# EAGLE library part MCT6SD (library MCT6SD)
Choice of 3 current transfer ratios; Two isolated channels per package; VDE approved for IEC60747-5-2; Two packages fit into a 16 lead DIP socket; Underwriters Laboratory (U.L.) recognized File E90700 Source: Datasheet
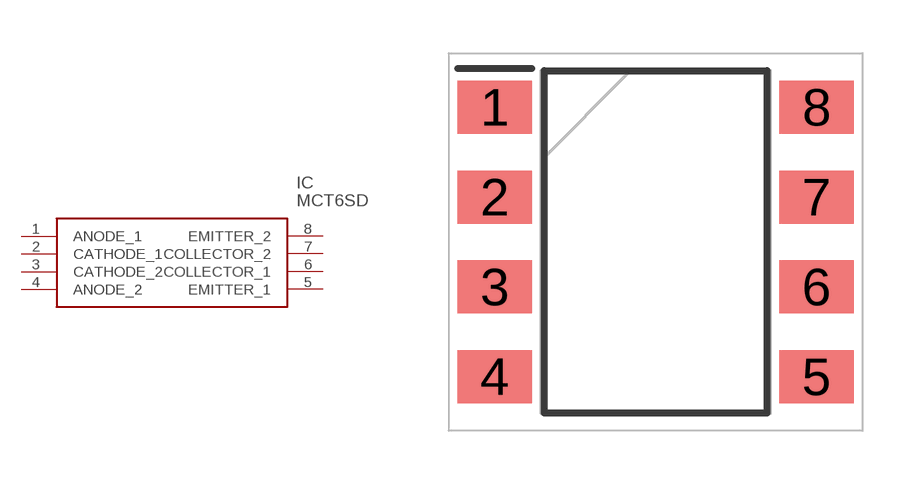
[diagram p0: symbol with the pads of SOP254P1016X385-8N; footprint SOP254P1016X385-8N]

Designator prefix IC

## MCT6SD (Description: Choice of 3 current transfer ratios; Two isolated channels per package; VDE approved for IEC60747-5-2; Two packages fit into a 16 lead DIP socket; Underwriters Laboratory (U.L.) recognized File E90700; Height: 3.85mm; Manufacturer_Name: onsemi; Manufacturer_Part_Number: MCT6SD; Mouser_Part_Number: 512-MCT6SD; Mouser_Price-Stock: https://www.mouser.co.uk/ProductDetail/onsemi-Fairchild/MCT6SD?qs=RjNHq7A%252BoByx0biQVmQP5w%3D%3D)  [SOP254P1016X385-8N]
1  ANODE_1
2  CATHODE_1
3  CATHODE_2
4  ANODE_2
5  EMITTER_1
6  COLLECTOR_1
7  COLLECTOR_2
8  EMITTER_2

## Footprint SOP254P1016X385-8N (pad centres in mm)
MCT6SD
smd 2.1 x 1.5: 1 -4.55,3.81; 2 -4.55,1.27; 3 -4.55,-1.27; 4 -4.55,-3.81; 5 4.55,-3.81; 6 4.55,-1.27; 7 4.55,1.27; 8 4.55,3.81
